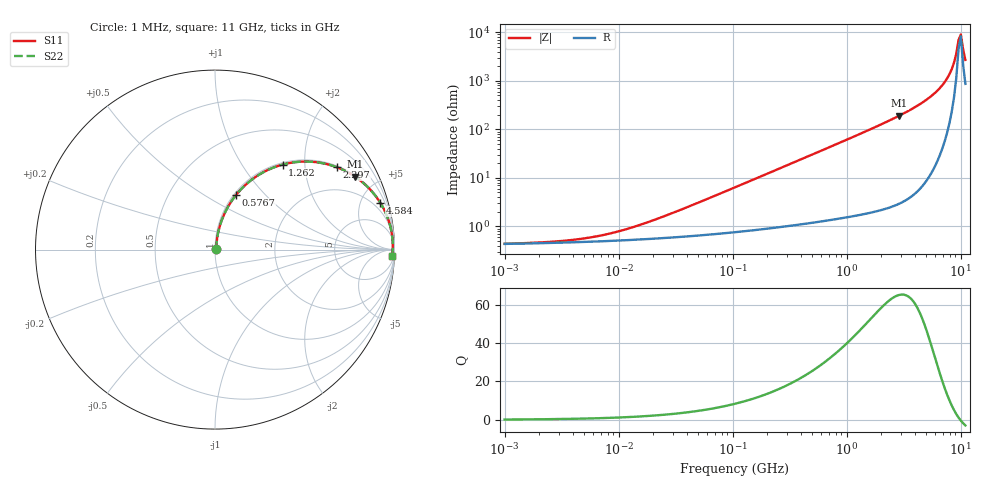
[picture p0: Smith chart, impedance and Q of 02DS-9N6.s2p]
# MHz S MA R 50
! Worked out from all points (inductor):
!   203 points, 1 MHz to 11 GHz, reference 50 ohm
!   read as one part in series: L = 9.6 nH near 30.23 MHz
!   highest Q = 65.1 at 2.892 GHz (marker M1), where L = 10.5 nH
!   self-resonance near 9.58 GHz
!   S11 on the Smith chart (normalised r, x): 1 MHz: 1.01, +0.00; 576.7 MHz: 1.02, +0.70; 1.262 GHz: 1.03, +1.55; 2.297 GHz: 1.05, +2.93; 4.584 GHz: 1.13, +7.04; 11 GHz: 18, -51
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1  0.004373 7.9  0.9957 -0.0  0.9957 -0.0  0.004373 7.9
4.78889  0.005547 31.1  0.9953 -0.2  0.9953 -0.2  0.005547 31.1
10.0079  0.007867 49.4  0.9949 -0.3  0.9949 -0.3  0.007867 49.4
22.9334  0.01487 66.9  0.9943 -0.8  0.9943 -0.8  0.01487 66.9
104.881  0.06312 79.6  0.9905 -3.6  0.9905 -3.6  0.06312 79.6
240.337  0.1425 78.1  0.9806 -8.2  0.9806 -8.2  0.1425 78.1
502.263  0.2877 71.1  0.9465 -16.7  0.9465 -16.7  0.2877 71.1
576.702  0.3261 68.9  0.9338 -19.0  0.9338 -19.0  0.3261 68.9
872.998  0.4637 60.8  0.8734 -27.6  0.8734 -27.6  0.4637 60.8
1262.03  0.6057 51.5  0.7825 -37.3  0.7825 -37.3  0.6057 51.5
2296.99  0.8197 34.0  0.5596 -55.0  0.5596 -55.0  0.8197 34.0
2405.28  0.833 32.7  0.5401 -56.4  0.5401 -56.4  0.833 32.7
2891.96  0.8802 27.5  0.4614 -61.6  0.4614 -61.6  0.8802 27.5
4584.18  0.9572 15.8  0.2718 -73.2  0.2718 -73.2  0.9572 15.8
6043.7  0.9803 9.7  0.1686 -78.5  0.1686 -78.5  0.9803 9.7
7609.17  0.9894 5.1  0.08831 -80.6  0.08831 -80.6  0.9894 5.1
8736.92  0.991 2.4  0.04227 -76.5  0.04227 -76.5  0.991 2.4
9148.82  0.9909 1.5  0.02755 -70.1  0.02755 -70.1  0.9909 1.5
9580.14  0.9906 0.6  0.01434 -48.6  0.01434 -48.6  0.9906 0.6
10031.8  0.9899 -0.3  0.011 23.2  0.011 23.2  0.9899 -0.3
10504.8  0.9889 -1.1  0.02242 59.8  0.02242 59.8  0.9889 -1.1
11000  0.9876 -2.0  0.03674 69.3  0.03674 69.3  0.9876 -2.0
